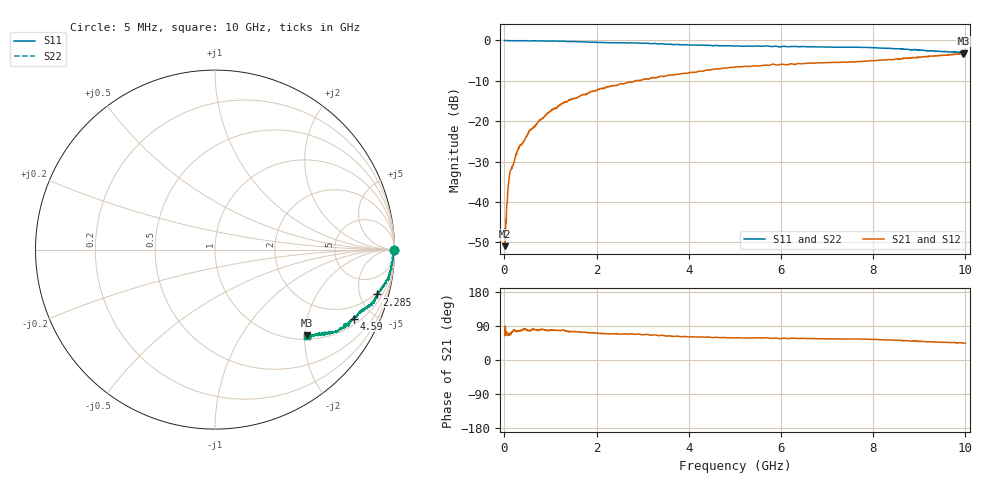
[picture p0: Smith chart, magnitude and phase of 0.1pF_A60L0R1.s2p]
! Amotech Co.,Ltd.
! http://www.amotech.co.kr/
! Part Number: A60L0R1
! These Parameters are Measured in Series Mode Connection
! Operation Temp=25[degC], DC Bias Voltage=0[V]
! Freq. Start=5[MHz] Stop=10[GHz], 2000[Steps]
! Date: Monday, July 14, 2020, 09:23:14
# GHZ S RI R 50.000000
!Freq.(Hz) S11(Real) S11(Imag) S21(Real) S21(Imag) S12(Real) S12(Imag) S22(Real) S22(Imag)
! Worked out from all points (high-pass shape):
!   2000 points, 5 MHz to 10 GHz, reference 50 ohm
!   highest |S21| = -3.28 dB at 9.94 GHz (marker M1); lowest = -51.0 dB at 10 MHz (marker M2)
!   |S21| within 3 dB of the highest: 5.518703 GHz to 5.529496 GHz (10.79 MHz wide, 0.195 % of centre); 5.532 GHz to end of sweep
!   lowest |S11| = -3.1 dB at 9.965 GHz (marker M3), VSWR 5.66, Z = 54.9 - j103 ohm
!   |S11| at or under -10 dB: nowhere
!   |S22| runs from -3.1 to 0.0 dB; largest |S21 - S12| = 1.1e-15
!   S11 on the Smith chart (normalised r, x): 5 MHz: open; 2.285 GHz: 1.72, -6.94; 4.59 GHz: 1.26, -3.89; 10 GHz: 1.09, -2.04
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0.005  0.9987 -0.00382  0.00132 0.00382  0.00132 0.00382  0.9987 -0.00382
0.01  0.9988 -0.00254  0.00125 0.00254  0.00125 0.00254  0.9988 -0.00254
0.04  0.9979 -0.00499  0.00214 0.00499  0.00214 0.00499  0.9979 -0.00499
0.095  0.9938 -0.0171  0.00622 0.0171  0.00622 0.0171  0.9938 -0.0171
0.125  0.9917 -0.022  0.0083 0.022  0.0083 0.022  0.9917 -0.022
0.15  0.9921 -0.0241  0.00787 0.0241  0.00787 0.0241  0.9921 -0.0241
0.265  0.9902 -0.0382  0.00976 0.0382  0.00976 0.0382  0.9902 -0.0382
0.325  0.9888 -0.0478  0.0112 0.0478  0.0112 0.0478  0.9888 -0.0478
0.56  0.9837 -0.0758  0.0163 0.0758  0.0163 0.0758  0.9837 -0.0758
0.945  0.9743 -0.123  0.0257 0.123  0.0257 0.123  0.9743 -0.123
1.275  0.968 -0.1645  0.032 0.1645  0.032 0.1645  0.968 -0.1645
1.675  0.9397 -0.2011  0.0603 0.2011  0.0603 0.2011  0.9397 -0.2011
2.285  0.902 -0.2497  0.098 0.2497  0.098 0.2497  0.902 -0.2497
3.34  0.8483 -0.3165  0.1517 0.3165  0.1517 0.3165  0.8483 -0.3165
4.59  0.7767 -0.3844  0.2233 0.3844  0.2233 0.3844  0.7767 -0.3844
5.005  0.7532 -0.3992  0.2468 0.3992  0.2468 0.3992  0.7532 -0.3992
6.67  0.7122 -0.4391  0.2878 0.4391  0.2878 0.4391  0.7122 -0.4391
7.645  0.6902 -0.4496  0.3098 0.4496  0.3098 0.4496  0.6902 -0.4496
8.335  0.6515 -0.4651  0.3485 0.4651  0.3485 0.4651  0.6515 -0.4651
9.94  0.5149 -0.4848  0.4851 0.4848  0.4851 0.4848  0.5149 -0.4848
9.965  0.5124 -0.4764  0.4876 0.4764  0.4876 0.4764  0.5124 -0.4764
10  0.5099 -0.4792  0.4901 0.4792  0.4901 0.4792  0.5099 -0.4792
